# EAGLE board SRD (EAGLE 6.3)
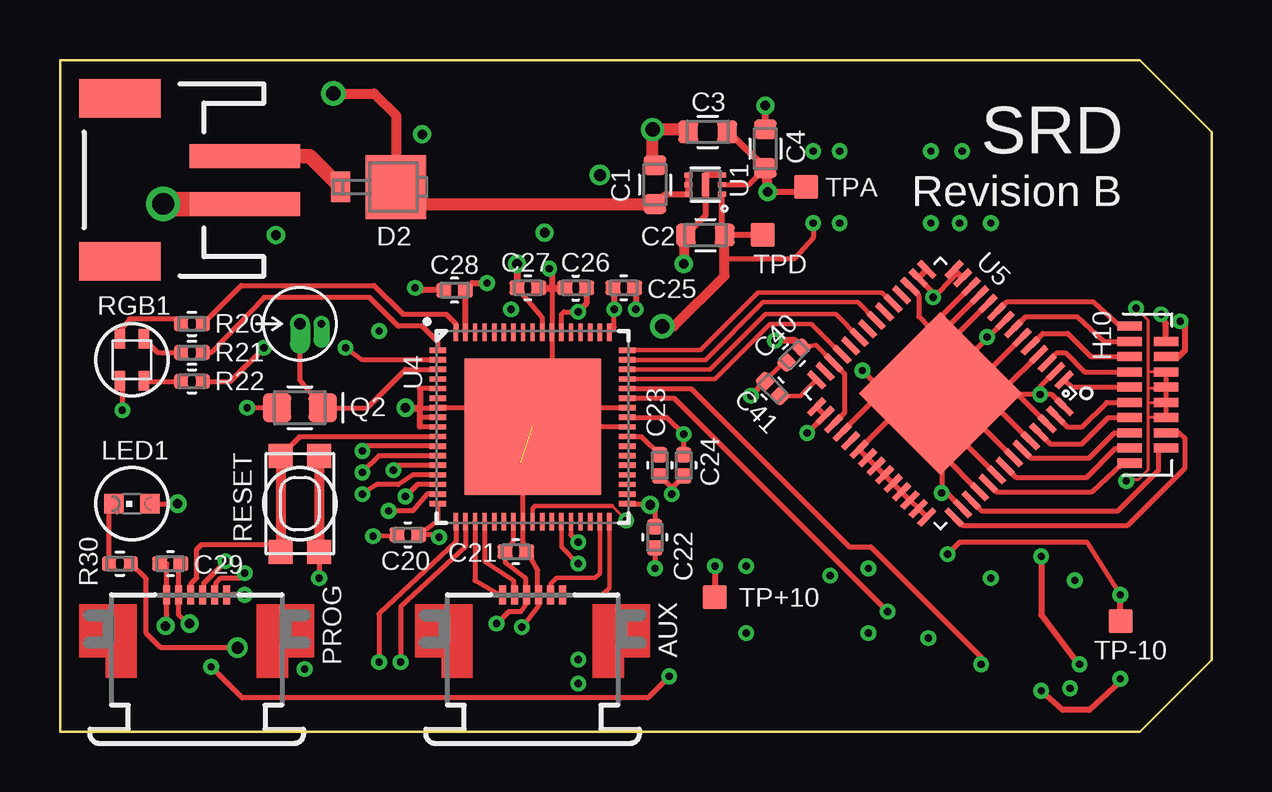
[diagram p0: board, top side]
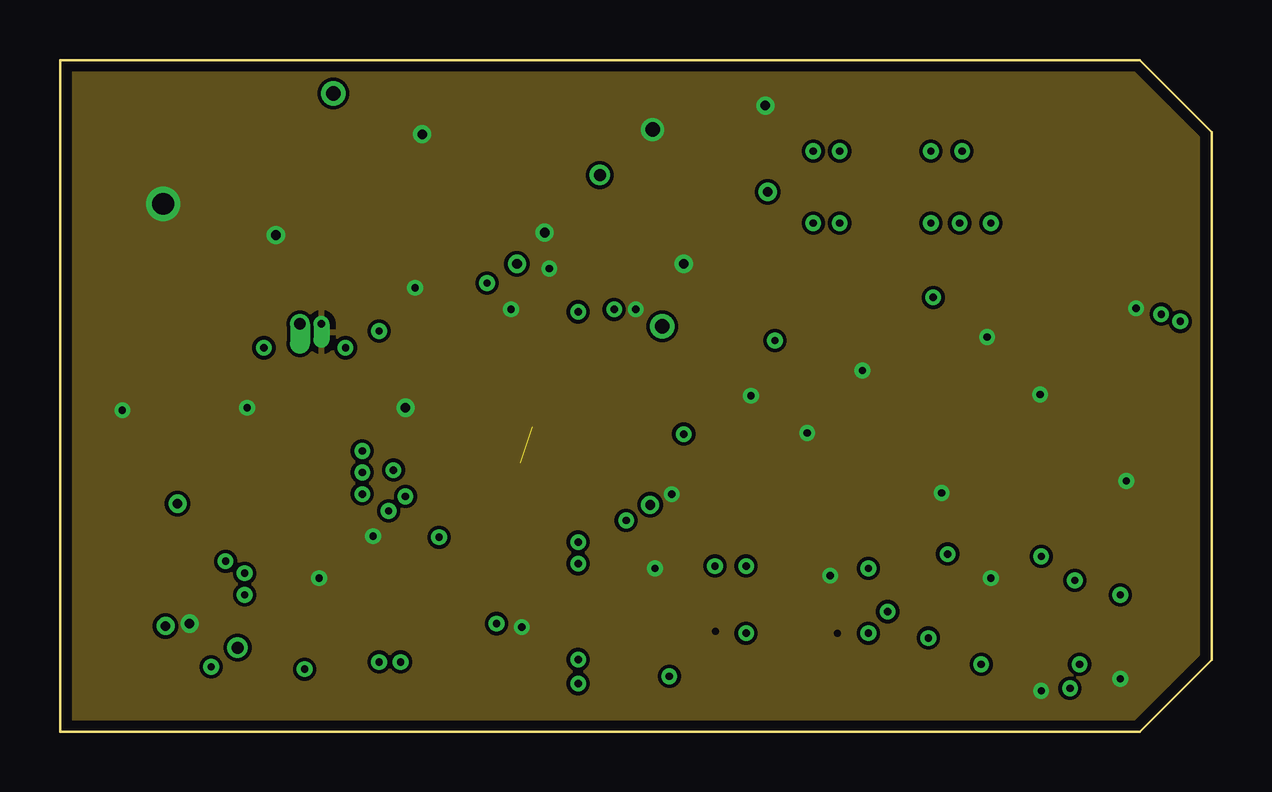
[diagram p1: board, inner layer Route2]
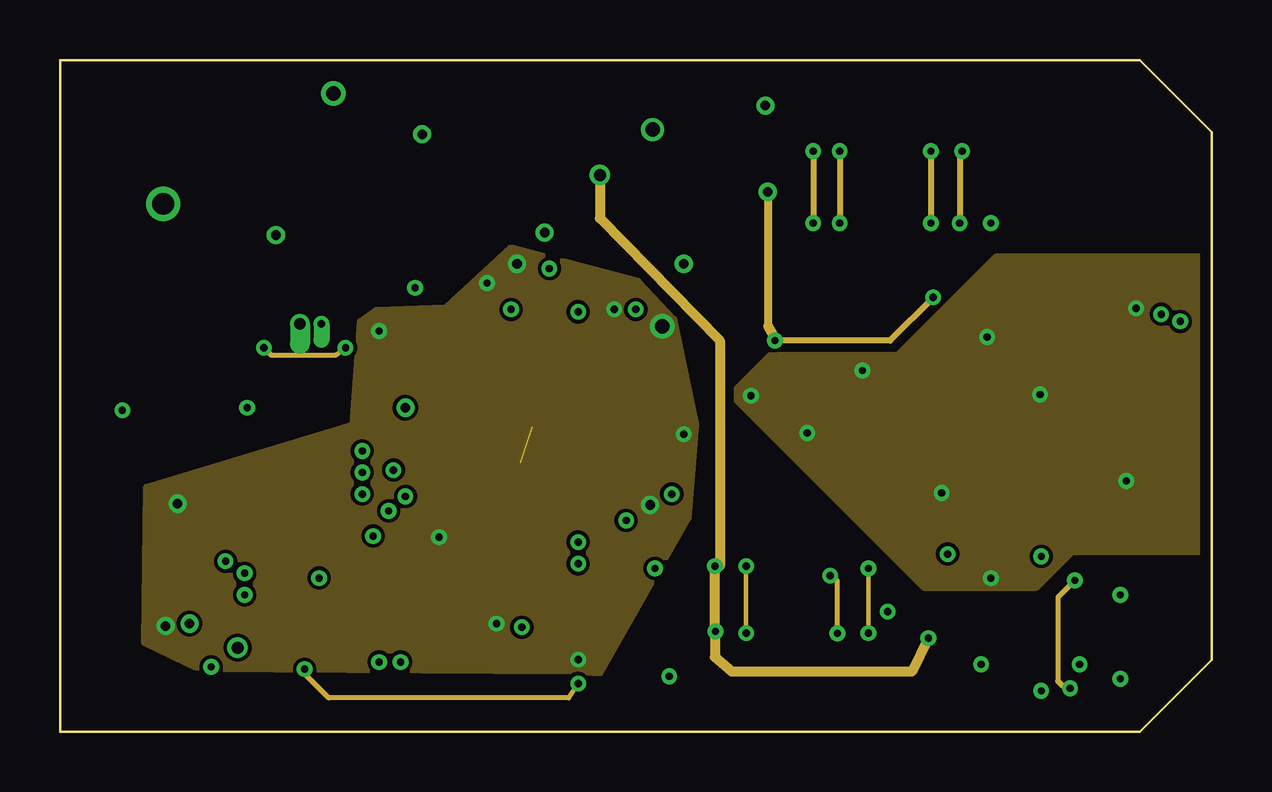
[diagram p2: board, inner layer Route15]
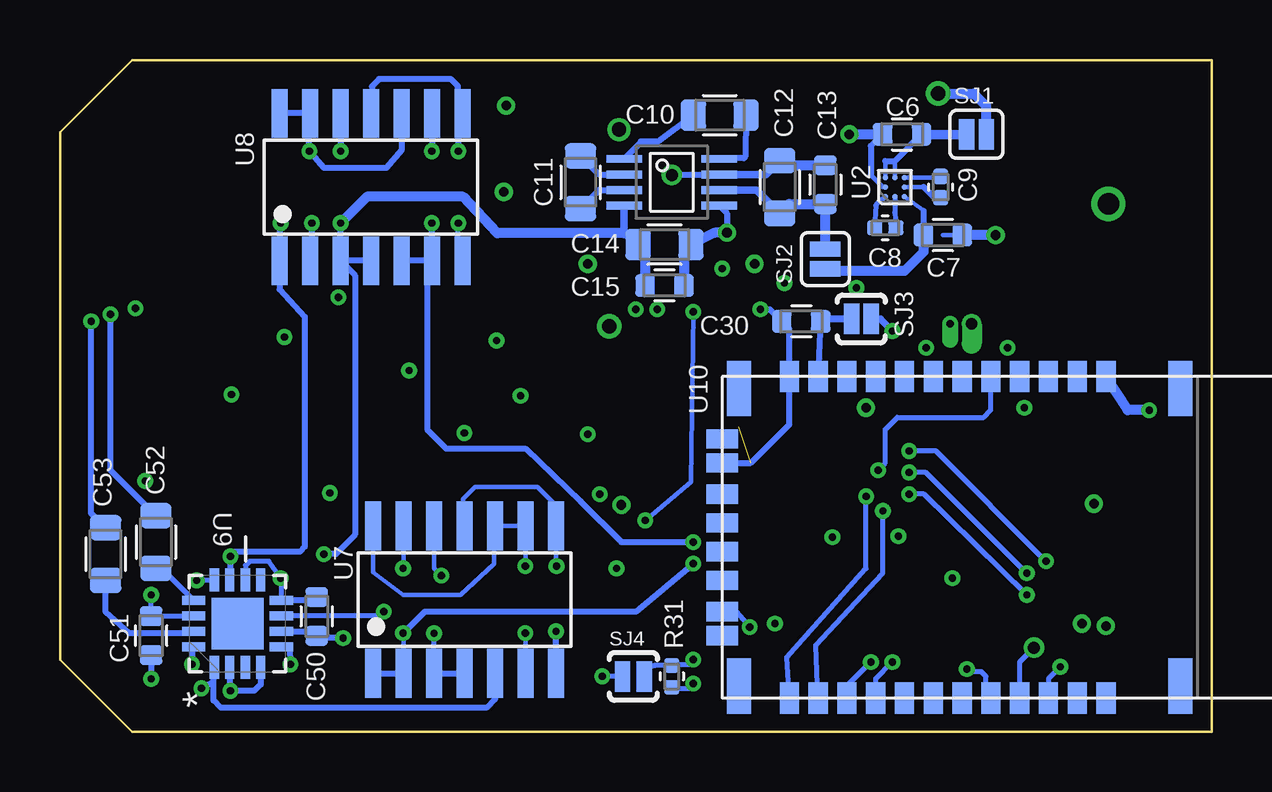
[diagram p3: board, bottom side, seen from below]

Size 48 x 28 mm. Coordinates in mm from the lower left corner, seen from the top.
Outline: 0,0 45,0 48,3 48,25 45,28 0,28 0,0
Copper layers ((1*2)+(15*16)): Top 0.0356mm / dielectric 1.5011mm / Route2 0.0356mm / dielectric 0.1499mm / Route15 0.0356mm / dielectric 0.2007mm / Bottom 0.0356mm
Design rules "LaenPCBOrder_johnmod": minimum track width 5mil, minimum drill 10mil, track to track 6mil, track to pad 6mil, pad to pad 6mil, via to via 6mil, smd to smd 6mil, copper to edge 17mil, drill to drill 6mil, minimum pad ring 7mil, minimum via ring 7mil, stop-mask expansion 0.04mm, vias tented up to drill 0.8mm, thermal gap 10mil

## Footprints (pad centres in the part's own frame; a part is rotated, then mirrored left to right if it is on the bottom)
52746-6 = smd 0.3 x 0.8: 1 -1.25,0.6; 2 -0.75,0.6; 3 -0.25,0.6; 4 0.25,0.6; 5 0.75,0.6; 6 1.25,0.6
JST-2-SMD = smd 1 x 4.6: 1 -1,-3.7; 2 1,-3.7 | smd 1.6 x 3.4: NC1 -3.4,1.5; NC2 3.4,1.5
CAPC1608X90N = smd 0.81 x 0.93: 1 -0.81,0; 2 0.81,0
CAPC1005X55N = smd 0.64 x 0.63: 1 -0.445,0; 2 0.445,0
CAPC2012X100N = smd 1.05 x 1.3: 1 -1.1,0; 2 1.1,0
DO-216AA = smd 0.8 x 1.27: A 0.7,0 | smd 2.54 x 2.67: C -1.6,0
OMNETCS-18PIN-SMD = smd 1.016 x 0.381: 1 1.524,5.715; 2 1.524,5.08; 3 1.524,4.445; 4 1.524,3.81; 5 1.524,3.175; 6 1.524,2.54; 7 1.524,1.905; 8 1.524,1.27; 9 1.524,0.635; 10 1.524,0; 11 0,0.635; 12 0,1.27; 13 0,1.905; 14 0,2.54; 15 0,3.175; 16 0,3.81; 17 0,4.445; 18 0,5.08
CHIPLED_0603 = smd 0.8 x 0.8: A 0,-0.75; C 0,0.75
MTD8000M3B-T = drill 0.47 pad 0.79 offset: C 0,0 | drill 0.32 pad 0.64 offset: E -0.9,0
OP501 = smd 1.2 x 1.2: C -0.955,0; E 0.955,0
RESC1005X35N = smd 0.59 x 0.6: 1 -0.455,0; 2 0.455,0
LED_RGB = smd 0.8 x 0.5: P$1 0.875,-0.5; P$2 -0.875,-0.5; P$3 -0.875,0.5; P$4 0.875,0.5
SJ_2S = smd 0.635 x 1.27: 1 -0.412,0; 2 0.412,0
SJ_2S-NOTRACE = smd 0.635 x 1.27: 1 -0.401,0; 2 0.413,0
SJ_2S-NO = smd 0.635 x 1.27: 1 -0.45,0; 2 0.45,0
KMR2 = smd 1 x 1: 1 2,0.8; 2 2,-0.8; 3 -2,0.8; 4 -2,-0.8
PAD1MMX1MM = smd 1 x 1: P$1 0,0
THIN_DFN = smd 0.35 x 0.18: P$1 -0.7,0.4; P$2 -0.7,0; P$3 -0.7,-0.4; P$4 0.7,-0.4; P$5 0.7,0; P$6 0.7,0.4 | smd 0.3 x 0.94: P$7 0,0
BGA9C40P3X3_121X121X63B27N = smd 0.22 x 0.22: A1 -0.4,-0.4; A2 -0.4,0; A3 -0.4,0.4; B1 0,-0.4; B3 0,0.4; C1 0.4,-0.4; C2 0.4,0; C3 0.4,0.4
UMAX8 = smd 1.5 x 0.3: P$1 -1.98,0.975; P$2 -1.98,0.325; P$3 -1.98,-0.325; P$4 -1.98,-0.975; P$5 1.98,-0.975; P$6 1.98,-0.325; P$7 1.98,0.325; P$8 1.98,0.975
QFN68_8MM_0.4PITCH = smd 0.7 x 0.2: P$1 -3.95,3.2; P$2 -3.95,2.8; P$3 -3.95,2.4; P$4 -3.95,2; P$5 -3.95,1.6; P$6 -3.95,1.2; P$7 -3.95,0.8; P$8 -3.95,0.4; P$9 -3.95,0; P$10 -3.95,-0.4; P$11 -3.95,-0.8; P$12 -3.95,-1.2; P$13 -3.95,-1.6; P$14 -3.95,-2; P$15 -3.95,-2.4; P$16 -3.95,-2.8; P$17 -3.95,-3.2; P$35 3.95,-3.2; P$36 3.95,-2.8; P$37 3.95,-2.4; P$38 3.95,-2; P$39 3.95,-1.6; P$40 3.95,-1.2; P$41 3.95,-0.8; P$42 3.95,-0.4; P$43 3.95,0; P$44 3.95,0.4; P$45 3.95,0.8; P$46 3.95,1.2; P$47 3.95,1.6; P$48 3.95,2; P$49 3.95,2.4; P$50 3.95,2.8; P$51 3.95,3.2 | smd 0.2 x 0.7: P$18 -3.2,-3.95; P$19 -2.8,-3.95; P$20 -2.4,-3.95; P$21 -2,-3.95; P$22 -1.6,-3.95; P$23 -1.2,-3.95; P$24 -0.8,-3.95; P$25 -0.4,-3.95; P$26 0,-3.95; P$27 0.4,-3.95; P$28 0.8,-3.95; P$29 1.2,-3.95; P$30 1.6,-3.95; P$31 2,-3.95; P$32 2.4,-3.95; P$33 2.8,-3.95; P$34 3.2,-3.95; P$52 3.2,3.95; P$53 2.8,3.95; P$54 2.4,3.95; P$55 2,3.95; P$56 1.6,3.95; P$57 1.2,3.95; P$58 0.8,3.95; P$59 0.4,3.95; P$60 0,3.95; P$61 -0.4,3.95; P$62 -0.8,3.95; P$63 -1.2,3.95; P$64 -1.6,3.95; P$65 -2,3.95; P$66 -2.4,3.95; P$67 -2.8,3.95; P$68 -3.2,3.95 | smd 5.7 x 5.7: P$69 0,0
QFN56_8_X_8_LARGE = smd 0.9 x 0.25: 1 -4.05,3.25; 2 -4.05,2.75; 3 -4.05,2.25; 4 -4.05,1.75; 5 -4.05,1.25; 6 -4.05,0.75; 7 -4.05,0.25; 8 -4.05,-0.25; 9 -4.05,-0.75; 10 -4.05,-1.25; 11 -4.05,-1.75; 12 -4.05,-2.25; 13 -4.05,-2.75; 14 -4.05,-3.25; 29 4.05,-3.25; 30 4.05,-2.75; 31 4.05,-2.25; 32 4.05,-1.75; 33 4.05,-1.25; 34 4.05,-0.75; 35 4.05,-0.25; 36 4.05,0.25; 37 4.05,0.75; 38 4.05,1.25; 39 4.05,1.75; 40 4.05,2.25; 41 4.05,2.75; 42 4.05,3.25 | smd 0.25 x 0.9: 15 -3.25,-4.05; 16 -2.75,-4.05; 17 -2.25,-4.05; 18 -1.75,-4.05; 19 -1.25,-4.05; 20 -0.75,-4.05; 21 -0.25,-4.05; 22 0.25,-4.05; 23 0.75,-4.05; 24 1.25,-4.05; 25 1.75,-4.05; 26 2.25,-4.05; 27 2.75,-4.05; 28 3.25,-4.05; 43 3.25,4.05; 44 2.75,4.05; 45 2.25,4.05; 46 1.75,4.05; 47 1.25,4.05; 48 0.75,4.05; 49 0.25,4.05; 50 -0.25,4.05; 51 -0.75,4.05; 52 -1.25,4.05; 53 -1.75,4.05; 54 -2.25,4.05; 55 -2.75,4.05; 56 -3.25,4.05 | smd 4.8 x 4.8: CENTER 0,0
SO14 = smd 2.032 x 0.66: 1 -3.073,4.445; 2 -3.073,3.175; 3 -3.073,1.905; 4 -3.073,0.635; 5 -3.073,-0.635; 6 -3.073,-1.905; 7 -3.073,-3.175; 8 3.073,-3.175; 9 3.073,-1.905; 10 3.073,-0.635; 11 3.073,0.635; 12 3.073,1.905; 13 3.073,3.175; 14 3.073,4.445
QFN65P400X400X100-17N = smd 0.965 x 0.381: 1 -1.829,0.965; 2 -1.829,0.33; 3 -1.829,-0.33; 4 -1.829,-0.965; 9 1.829,-0.965; 10 1.829,-0.33; 11 1.829,0.33; 12 1.829,0.965 | smd 0.381 x 0.965: 5 -0.965,-1.829; 6 -0.33,-1.829; 7 0.33,-1.829; 8 0.965,-1.829; 13 0.965,1.829; 14 0.33,1.829; 15 -0.33,1.829; 16 -0.965,1.829 | smd 2.159 x 2.159: 17 0,0
RN42 = smd 1.3 x 0.8: 1 -6.7,6; 2 -6.7,4.8; 3 -6.7,3.6; 4 -6.7,2.4; 5 -6.7,1.2; 6 -6.7,0; 7 -6.7,-1.2; 8 -6.7,-2.4; 9 -6.7,-3.6; 10 -6.7,-4.8; 11 -6.7,-6; 12 -6.7,-7.2; 13 6.7,-7.2; 14 6.7,-6; 15 6.7,-4.8; 16 6.7,-3.6; 17 6.7,-2.4; 18 6.7,-1.2; 19 6.7,0; 20 6.7,1.2; 21 6.7,2.4; 22 6.7,3.6; 23 6.7,4.8; 24 6.7,6 | smd 0.8 x 1.3: 28 3.1,-10; 29 -3.1,-10; 30 4.1,-10; 31 1.8,-10; 32 0.6,-10; 33 -0.6,-10; 34 -1.8,-10; 35 -4.1,-10 | smd 2.3 x 1: SH1 -6.2,9.1; SH2 -6.2,-9.3; SH3 6.2,-9.3; SH4 6.2,9.1

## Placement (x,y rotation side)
AUX  52746-6  [52746-6]  19.7,5.1 0 top
BAT  M02-JST-2MM-SMT  [JST-2-SMD]  4,23 90 top
C1  1uF  [CAPC1608X90N]  24.8,22.8 90 top
C2  1uF  [CAPC1608X90N]  26.9,20.7 180 top
C3  1uF  [CAPC1608X90N]  27,25 180 top
C4  1uF  [CAPC1608X90N]  29.4,24.3 90 top
C6  2.2uF  [CAPC1608X90N]  12.9,24.9 180 bottom
C7  2.2uF  [CAPC1608X90N]  11.2,20.7 0 bottom
C8  220nF  [CAPC1005X55N]  13.6,21 0 bottom
C9  220nF  [CAPC1005X55N]  11.3,22.7 90 bottom
C10  3.3uF  [CAPC2012X100N]  20.5,25.7 180 bottom
C11  3.3uF  [CAPC2012X100N]  26.3,22.9 90 bottom
C12  3.3uF  [CAPC2012X100N]  18,22.7 90 bottom
C13  1uF  [CAPC1608X90N]  16.1,22.8 90 bottom
C14  3.3uF  [CAPC2012X100N]  22.8,20.3 0 bottom
C15  1uF  [CAPC1608X90N]  22.8,18.6 0 bottom
C20  0.1uF  [CAPC1005X55N]  14.5,8.2 180 top
C21  0.1uF  [CAPC1005X55N]  19,7.5 0 top
C22  0.1uF  [CAPC1005X55N]  24.8,8.1 270 top
C23  1uF  [CAPC1005X55N]  25,11.1 270 top
C24  0.1uF  [CAPC1005X55N]  26,11.1 90 top
C25  0.1uF  [CAPC1005X55N]  23.5,18.5 0 top
C26  0.1uF  [CAPC1005X55N]  21.5,18.5 180 top
C27  1uF  [CAPC1005X55N]  19.5,18.5 0 top
C28  0.1uF  [CAPC1005X55N]  16.45,18.4 0 top
C29  0.1uF  [CAPC1005X55N]  4.6,7 0 top
C30  [CAPC1608X90N]  17.1,17.1 0 bottom
C40  100nF  [CAPC1005X55N]  30.6,15.7 225 top
C41  10nF  [CAPC1005X55N]  29.7,14.3 135 top
C50  0.1uF  [CAPC1608X90N]  37.3,4.8 90 bottom
C51  0.1uF  [CAPC1608X90N]  44.2,4 270 bottom
C52  [CAPC2012X100N]  44,7.9 90 bottom
C53  [CAPC2012X100N]  46.1,7.4 90 bottom
D2  DIODE  [DO-216AA]  12.4,22.7 180 top
H10  A79043-001  [OMNETCS-18PIN-SMD]  46.1,16.9 180 top
LED1  [CHIPLED_0603]  3,9.5 90 top
PROG  52746-6  [52746-6]  5.7,5.1 0 top
Q1  [MTD8000M3B-T]  10,17 180 top
Q2  PHOTOTRANSISTOR_D  [OP501]  10,13.5 180 top
R20  1k  [RESC1005X35N]  5.5,17 180 top
R21  1k  [RESC1005X35N]  5.5,15.8 180 top
R22  1k  [RESC1005X35N]  5.5,14.6 180 top
R30  1k  [RESC1005X35N]  2.5,7 180 top
R31  1k  [RESC1005X35N]  22.5,2.3 90 bottom
RGB1  LED_RGB  [LED_RGB]  3,15.5 270 top
SJ1  SOLDERJUMPERNC  [SJ_2S]  9.8,24.9 0 bottom
SJ2  SOLDERJUMPERNC  [SJ_2S]  16.1,19.7 90 bottom
SJ3  SOLDERJUMPERNC2  [SJ_2S-NOTRACE]  14.6,17.2 0 bottom
SJ4  SOLDERJUMPERNO  [SJ_2S-NO]  24.1,2.3 0 bottom
SW1  SPST_TACT-KMR2  [KMR2]  10,9.5 270 top
TP+10  TEST-POINT  [PAD1MMX1MM]  27.3,5.6 0 top
TP-10  TEST-POINT  [PAD1MMX1MM]  44.2,4.6 0 top
TPA  TEST-POINT  [PAD1MMX1MM]  31.1,22.7 0 top
TPD  TEST-POINT  [PAD1MMX1MM]  29.3,20.7 0 top
U1  MIC5392/3  [THIN_DFN]  26.9,22.8 180 top
U2  AS1302BGA  [BGA9C40P3X3_121X121X63B27N]  13.2,22.7 0 bottom
U3  MAX865  [UMAX8]  22.5,22.9 0 bottom
U4  CY8C3866  [QFN68_8MM_0.4PITCH]  19.7,12.7 0 top
U5  RHD2216_QFN  [QFN56_8_X_8_LARGE]  36.7,14.1 225 top
U7  ALD1105  [SO14]  30.5,5.5 90 bottom
U8  ALD1105  [SO14]  34.4,22.7 90 bottom
U9  DG9409DN-T1-E4  [QFN65P400X400X100-17N]  40.6,4.5 90 bottom
U10  RN42  [RN42]  10.4,8.1 270 bottom

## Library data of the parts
AUX PROG = con-molex; OC_FARNELL: unknown; OC_NEWARK: unknown
BAT = SparkFun-Connectors; PROD_ID: CONN-08352
C1-C4 C6-C15 C20-C30 C40 C41 C50-C53 D2 H10 LED1 Q1 Q2 R20-R22 R30 R31 RGB1 SJ1-SJ4 TP+10 TP-10 TPA TPD U2 U7 U8 U10 = Ramshur
SW1 = _adafruit
U1 U3 U4 = _ramshur
U5 = RHD2000
U9 = DG9409; MPN: DG9409DN-T1-E4; OC_FARNELL: -; OC_NEWARK: 65K2483; PACKAGE: QFN-16; SUPPLIER: VISHAY SILICONIX

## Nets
5VDD: C7.1 SJ2.1 U2.C1
+10VDD: C12.2 C13.2 C50.1 TP+10.P$1 U3.P$7 U7.7 U7.8 U7.11 U9.6
-10VDD: C14.1 C15.1 C51.1 TP-10.P$1 U3.P$4 U8.3 U8.4 U8.12 U9.14
AUX_A1: AUX.5 U4.P$33
AUX_A2: AUX.6 U4.P$34
AUX_D1: AUX.1 U4.P$20
AUX_D2: AUX.2 U4.P$21
AVDD: C3.1 C4.1 C40.1 TPA.P$1 U1.P$2 U5.13 U5.14 U5.15 U5.16 U5.26 U5.31
CH0+: H10.10 U5.9
CH1+: H10.9 U5.7
CH2+: H10.8 U5.5
CH3+: H10.7 U5.3
CH4+: H10.6 U5.1
CH5+: H10.5 U5.55
CH6+: H10.4 U5.53
CH7+: H10.3 U5.51
CH8+: H10.2 U5.49
CH9+: H10.1 U5.47
CH10+: H10.18 U5.45
CH11+: H10.17 U5.43
DVDD: AUX.3 C2.1 C20.1 C21.1 C22.1 C24.2 C25.1 C27.1 C28.2 C29.1 LED1.A PROG.1 R31.2 SJ3.2 SJ4.2 TPD.P$1 U1.P$1 U4.P$17 U4.P$24 U4.P$35 U4.P$44 U4.P$52 U4.P$59 U4.P$67 U8.7 U8.8 U8.11
GND: AUX.4 BAT.1 C1.2 C2.2 C3.2 C4.2 C6.2 C7.2 C14.2 C15.2 C20.2 C21.2 C22.2 C23.2 C24.1 C25.2 C26.2 C27.2 C28.1 C29.2 C30.1 C40.2 C41.2 C50.2 C51.2 H10.13 H10.14 H10.15 H10.16 PROG.2 Q1.E Q2.E RGB1.P$1 SW1.1 SW1.3 U1.P$3 U1.P$7 U2.A2 U3.P$5 U4.P$5 U4.P$7 U4.P$8 U4.P$9 U4.P$25 U4.P$43 U4.P$45 U4.P$58 U4.P$69 U5.2 U5.4 U5.6 U5.8 U5.10 U5.11 U5.12 U5.17 U5.29 U5.30 U5.32 U5.34 U5.35 U5.36 U5.37 U5.38 U5.39 U5.40 U5.41 U5.42 U5.44 U5.46 U5.48 U5.50 U5.52 U5.54 U5.56 U5.CENTER U7.3 U7.4 U7.12 U9.2 U9.4 U9.8 U9.10 U10.1 U10.12 U10.28 U10.29
IDAC1: U4.P$29 U7.1 U7.2 U7.13
IDAC2: U4.P$30 U8.5 U8.6 U8.9
ISTIM+: U7.5 U9.1 U9.12
ISTIM-: U8.1 U9.11 U9.16
LED1: R20.1 U4.P$68
LED2: R21.1 U4.P$1
LED3: R22.1 U4.P$2
MISO: U4.P$48 U5.25
MOSI: U4.P$49 U5.23
N$1: C12.1 C13.1 SJ2.2 U3.P$6
N$2: C41.1 U5.28
N$3: R20.2 RGB1.P$2
N$4: C6.1 SJ1.1 U2.A3 U2.B3
N$5: R21.2 RGB1.P$3
N$6: C52.1 U9.13
N$7: R22.2 RGB1.P$4
N$8: LED1.C R30.2
N$9: C30.2 SJ3.1 U10.11
N$11: U7.6 U7.9 U7.10 U7.14
N$17: C53.1 U9.15
N$30: C23.1 U4.P$42
N$31: U8.2 U8.10 U8.13 U8.14
N$33: C8.1 U2.A1
N$36: C9.2 U2.C3
N$42: C11.1 U3.P$3
N$46: C11.2 U3.P$2
N$47: C10.1 U3.P$8
N$48: C10.2 U3.P$1
N$49: C8.2 U2.B1
N$50: C9.1 U2.C2
PIO2: U10.19
PIO3: R31.1 U10.20
PIO4: SJ4.1 U10.22
PIO5: R30.1 U10.21
RN_RESET: U4.P$13 U10.5
SCLK: U4.P$50 U5.21
SS: U4.P$51 U5.19
STIME1: C52.2 H10.11
STIME2: C53.2 H10.12
STIMSEL0: U4.P$46 U9.7
STIMSEL1: U4.P$47 U9.5
SWDCK: PROG.5 U4.P$12
SWDIO: PROG.4 U4.P$11
SWV: PROG.6 U4.P$14
SYNC: Q1.C Q2.C U4.P$3
UART_CTS: U4.P$18 U10.16
UART_RTS: U4.P$19 U10.15
UART_RX: U4.P$16 U10.14
UART_TX: U4.P$15 U10.13
VBAT: BAT.2 D2.A
VCCD: C26.1 U4.P$26 U4.P$57
VIN: C1.1 D2.C SJ1.2 U1.P$4 U1.P$5 U1.P$6
XRES: PROG.3 SW1.2 SW1.4 U4.P$10

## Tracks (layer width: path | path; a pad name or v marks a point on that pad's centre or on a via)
5VDD
  Bottom 0.178: 12,21.71 U2.C1
  Bottom 0.254: C7.1 12,21.71
  Bottom 0.406: C7.1 12.01,19.99 12.8,19.2 16.09,19.2 SJ2.1
+10VDD  (via drill 0.3, 0.3 layers 15-16, 0.5)
  Top 0.254: v27.3,6.9 TP+10.P$1
  Route15 0.406: v22.5,23.2 22.5,21.4 27.5,16.3 27.5,6.9 v27.3,6.9 27.3,4.2 v27.32,4.17 27.3,4.15 27.3,3.1 28,2.5 35.5,2.5 v36.2,3.9
  Bottom 0.178: U7.11 31.2,8.64 31.2,9.7 30.7,10.2 28.1,10.2 27.32,9.43 U7.8 27.32,6.92 v27.3,6.9
  Bottom 0.254: v22.5,23.2 22.18,23.23 U3.P$7 | U9.6 37.48,4.17 C50.1 | 37.29,3.8 C50.1 | v36.2,3.9 37.21,3.9 C50.1 | U7.7 v27.32,4.17
  Bottom 0.305: C12.2 18.57,23.23 U3.P$7
  Bottom 0.406: C12.2 17.81,23.61 C13.2
-10VDD  (via drill 0.3)
  Top 0.2: v37,7.4 37.5,7.9 42.8,7.9 v44.2,5.7
  Top 0.254: TP-10.P$1 v44.2,5.7
  Route15 0.254: v36.3,24.2 v36.3,21.2
  Bottom 0.2: v44.2,5.7 C51.1 43.92,4.83 U9.14
  Bottom 0.254: U8.4 U8.3 | U8.12 v36.3,24.2 | U8.3 35.7,19.02 35.7,8.2 36.5,7.4 v37,7.4 | U8.3 v36.3,21.2 | U9.14 42.49,4.89
  Bottom 0.305: C14.1 24.32,20.64 24.48,20.78 U3.P$4
  Bottom 0.406: C14.1 23.61,20.01 C15.1 | 35,19.36 U8.4 | 24.48,20.78 29.78,20.78 31.2,22.3 35.2,22.3 v36.3,21.2
AUX_A1
  Top 0.178: U4.P$33 22.5,6.6 22.3,6.4 20.7,6.4 20.45,6.15 AUX.5
AUX_A2
  Top 0.178: U4.P$34 22.9,6 22.6,5.7 AUX.6
AUX_D1
  Top 0.2: U4.P$20 17.3,6.3 18.4,5.65 AUX.1
AUX_D2
  Top 0.2: U4.P$21 17.7,7.1 18.9,6.3 18.9,5.65 AUX.2
AVDD  (via drill 0.3, 0.4)
  Top 0.178: C40.1 31.5,16.11 U5.26
  Top 0.2: U5.16 36.4,18.29 v36.4,18.1 37.27,18.97 U5.14 | U1.P$2 28.71,22.8 C4.1 | U5.26 32.7,14.92 32.7,13.28 U5.31
  Top 0.254: U5.16 U5.15 | U5.13 U5.14 | TPA.P$1 30.9,22.5 v29.5,22.5
  Top 0.3: C4.1 27.89,25 C3.1 | C40.1 30.63,16.3 v29.8,16.3
  Top 0.406: C4.1 v29.5,22.5
  Route15 0.254: v36.4,18.1 34.6,16.3 v29.8,16.3
  Route15 0.3: 29.8,16.4 v29.8,16.3
  Route15 0.34: v29.5,22.5 29.5,16.9
  Route15 0.4: 29.5,16.9 29.8,16.4
CH0+
  Top 0.2: U5.9 39.44,17.9 43.1,17.9 44.2,16.9 H10.10
CH1+
  Top 0.2: U5.7 40.25,17.3 42.4,17.3 43.53,16.27 H10.9
CH2+
  Top 0.2: U5.5 40.97,16.6 42,16.6 42.97,15.63 H10.8
CH3+
  Top 0.2: U5.3 41.58,15.8 41.9,15.8 42.7,14.99 H10.7
CH4+
  Top 0.2: U5.1 42.17,14.36 H10.6
CH5+
  Top 0.2: U5.55 41.99,12.7 42.6,12.7 43.62,13.72 H10.5
CH6+
  Top 0.2: U5.53 41.27,12 42.6,12 43.69,13.09 H10.4
CH7+
  Top 0.2: U5.51 40.46,11.4 42.9,11.4 43.95,12.46 H10.3
CH8+
  Top 0.2: U5.49 39.85,10.6 42.8,10.6 44.02,11.82 H10.2
CH9+
  Top 0.2: U5.47 39.03,10 43,10 44.28,11.19 H10.1
CH10+
  Top 0.2: U5.45 38.42,9.2 44.1,9.2 45.8,10.9 45.8,11.6 45.82,11.82 H10.18
CH11+
  Top 0.2: U5.43 37.6,8.6 44.5,8.6 46.9,11 46.9,12.2 46.65,12.46 H10.17
DVDD  (via drill 0.3, 0.4, 0.6 pad 1.02)
  Top 0.2: U4.P$24 18.9,7.95 C21.1 18.55,7.04 19.4,6.4 19.4,5.65 AUX.3 19.45,5.35 19.2,5 18.7,5 v18.2,4.5 | C20.1 15.75,8.79 U4.P$17 | v4.4,4.4 4.45,4.85 PROG.1 4.45,7 C29.1 | C20.1 15.1,8.04 15.15,8.04 | LED1.A v4.9,9.5 | C27.1 20.1,17.25 U4.P$59 | v15.8,8.1 15.7,8.21 C20.1 | U4.P$52 23.1,16.85 v23.1,17.6 | v31.4,21.2 31.4,20.6 30.6,19.7 27.7,19.7 | C24.2 v26,12.4 25.3,13.1 U4.P$44 | U4.P$35 24.6,9.5 v24.6,9.45 24.8,9.25 C22.1
  Top 0.254: U1.P$1 27.6,20.7 C2.1 TPD.P$1 | U4.P$67 C28.2 17.2,18.7 v17.8,18.7 | C25.1 23.1,18.45 v23.1,17.6
  Top 0.3: v19.05,19.5 C27.1
  Top 0.406: C2.1 27.7,19.7 27.7,19 25.6,16.9 v25.1,16.9
  Route15 0.254: v31.4,24.2 v31.4,21.2
  Bottom 0.2: SJ4.2 arc90 23.2,2.75 R31.2 arc90 22.45,2.8 21.8,2.8 v21.6,3 | 31.4,19.63 v31.4,21.2
  Bottom 0.254: v31.4,24.2 31.4,25.77 U8.8 31.43,26.93 31.7,27.2 34.7,27.2 35,26.9 35,25.74 U8.11 | U8.7 31.4,19.63
  Bottom 0.3: SJ3.2 13.8,17.2 v13.3,16.7
  pour Route15: 24.1,18.8 25.6,17.2 26.5,12.8 26.2,8.9 22.5,2.4 21.2,2.5 5.8,2.6 3.5,3.7 3.6,10.2 12.2,12.8 12.5,17.1 13.2,17.6 16.1,17.7 18.8,20.2
GND  (via drill 0.3, 0.3 layers 15-16, 0.4, 0.6, 0.9 pad 1.42)  (1 unrouted)
  Top 0.127: v44.85,17.65 45.35,17.15 45.35,15 | 45.35,15 45.35,14.3 | 45.35,14.3 45.35,10.9 44.95,10.5 44.5,10.5 | H10.13 45.35,15 | H10.14 46.04,14.3 45.35,14.3 | 46.1,13.7 45.4,13.7 | H10.16 45.4,13.1
  Top 0.178: 21.8,13.4 21.8,12.9 22,12.7 | C40.2 30.18,15.41 C41.2
  Top 0.2: v5.4,4.5 4.95,4.85 PROG.2 4.95,6.8 C29.2 | C20.2 14,8.14 v13.05,8.15 | 15,13.5 U4.P$7 17.4,13.5 | U4.P$8 15,13.1 | U4.P$9 15,12.7 | U4.P$5 15,14.3 | U5.42 U5.41 U5.40 U5.39 U5.38 U5.37 U5.36 U5.35 U5.34 35.04,13.5 35.1,13.5 | U5.29 U5.30 31.16,12.45 v31.15,12.45 | RGB1.P$1 2.6,14.53 v2.6,13.4 | U5.12 36.8,17.38 36.8,17.1 | U5.11 36.9,16.77 36.9,16.4 37.23,16.4 | U5.10 37.23,16.4 | 37.7,15.4 37.7,15.45 U5.8 37.95,15.7 37.7,15.7 37.23,16.17 37.23,16.4 | U5.6 38.5,14.84 38.5,14.7 | U5.4 39.38,14.3 | 39.38,14.3 39.2,14.3 | U5.54 39.68,14.3 39.38,14.3 | U5.56 41.35,14.05 v40.85,14.05 | v40.85,14.05 38.9,14.05 38.45,14.05 | U5.52 39.07,13.5 39,13.5 | U5.50 38.1,13.05 | 38.1,13.05 38.1,13.3 | U5.48 37.6,12.14 | 37.6,12.14 37.6,12.9 | U5.46 36.8,11.53 36.8,11.8 36.75,11.75 v36.75,9.95 36.96,9.95 U5.44 | 38.1,13.05 37.73,13.43 37.05,14.1 U5.CENTER | 37.6,12.14 37.6,11.82 | SW1.1 v10.8,6.4 | Q2.E v7.8,13.5 | 20.5,14.8 U4.P$58 20.5,18.5 | 20.5,14.8 20.4,14.8 | U4.P$43 22,12.7 | 19.3,10.7 U4.P$25 19.3,7.9 19.9,6.7 | U4.P$45 21.9,13.5 arc90 21.8,13.4 21.8,14.8 20.5,14.8 | v19.25,4.35 19.95,5.25 AUX.4 19.95,5.95 19.9,6 | C21.2 19.9,6.75 19.9,6.7 | 19.9,5.7 19.9,6 | 19.9,6 19.9,6.7 | U5.17 35.8,18.18 35.8,17.3 36.23,16.88 36.8,16.88 | U5.32 32.6,12.5 34.2,14.1 34.2,14.3 v33.45,15.05 | U5.2 40.85,14.36 v40.85,14.05 | H10.13 H10.14 H10.15 46.1,13.7 H10.16 | C22.2 v24.8,6.8 | C23.2 25.5,10.15 | C24.1 25.5,10.15 | 25.5,10.15 v25.5,9.9
  Top 0.25: 15,12.7 15,13.1 15,13.5 15,14.3
  Top 0.254: U1.P$3 26.9,23.2 U1.P$7 26.9,21.51 C2.2 26,20.61 | C1.2 24.7,23.71 | C3.2 26.09,25.1 | C41.2 29.39,14.59 v28.8,14 | 37.7,15.4 38.26,14.84 38.5,14.84 | 37.73,13.33 38.4,14 38.5,14 38.45,14.05 38.7,14.3 | 37.6,12.9 37.6,13.2 37.73,13.33 | 37.73,13.33 37.73,13.43 | 39,13.5 38.9,13.6 38.9,14.05 | 38.7,14.3 39.2,14.3 | 38.7,14.3 38.5,14.5 38.5,14.7 | 36.9,16.77 36.8,16.88 36.8,17.1 | U5.CENTER 36.1,13.5 35.1,13.5 | C28.1 15.1,18.4 v14.8,18.5 | v20.4,19.3 20.5,19.2 20.5,18.5 | C25.2 24,18.45 v24,17.6 | v44.2,2.2 44.2,2.1 42.9,0.9 41.8,0.9 v40.9,1.7
  Top 0.3: C27.2 20.5,18.5 C26.2 | v14.4,13.5 15,13.5 | C4.2 v29.4,26.1
  Top 0.406: SW1.3 SW1.1 | 26,20.61 v26,19.5
  Top 0.5: 24.7,23.71 v24.7,25.1 26.09,25.1
  Top 1.016: BAT.1 v4.3,22
  Route15 0.2: v32.41,4.09 32.41,6.29 v32.1,6.5
  Bottom 0.178: 14.2,23.2 13.7,22.7 U2.A2 | C7.2 11.19,20.7 | U7.12 32.41,6.8 v32.1,6.5
  Bottom 0.2: U10.28 19.8,5 v19.25,4.35 | U7.3 v32.41,4.09 | U9.8 38.77,6.37 v38.8,6.4 39.3,7.1 40.1,7.1 40.27,6.93 U9.10
  Bottom 0.254: C6.2 14.2,24.41 14.2,23.2 | U7.3 U7.4 | U9.2 40.9,2.64 v40.9,1.7 39.9,1.7 39.63,1.97 U9.4 | C50.2 37.65,5.46 U9.8 | U3.P$5 20.2,21.61 v20.2,20.8 | C51.2 v44.2,2.2 | v18.8,17.6 18.41,17.6 C30.1 17.6,16.79 U10.12 17.6,12.8 19.2,11.2 U10.29
  Bottom 0.406: v15.1,24.9 C6.2 | v9,20.7 C7.2 | C15.2 21.99,20.11 C14.2 20.7,20.8 v20.2,20.8 | v2.6,13.4 3.5,13.4 U10.1
  other vias: 38.65,16.45 44.45,10.45
  pour Route2: 0.2,0.2 47.8,0.2 47.8,27.9 0.2,27.8
  pour Route15: 47.8,19.8 39,19.8 34.9,15.7 29.6,15.7 28.2,14.3 28.2,13.8 36,6 40.7,6 42.2,7.5 47.8,7.5
IDAC1  (via drill 0.3)
  Top 0.178: U4.P$29 20.9,7.7 v21.6,7
  Route15 0.178: v33.7,6.8 v33.7,4.1
  Bottom 0.178: U7.2 33.67,4.08 v33.7,4.1 | U7.13 33.67,6.83 v33.7,6.8
  Bottom 0.254: U7.1 U7.2 | v21.6,7 24,5 32.8,5 v33.7,4.1
IDAC2  (via drill 0.3)
  Top 0.178: U4.P$30 21.3,8.2
  Top 0.2: 21.3,8.2 v21.6,7.9
  Route15 0.254: v32.5,24.2 v32.5,21.2
  Bottom 0.254: U8.6 U8.5 | U8.9 v32.5,24.2 | U8.6 32.7,19.09 32.7,12.6 31.9,11.8 28.6,11.8 26.3,9.6 24.6,7.9 v21.6,7.9 | U8.6 v32.5,21.2
ISTIM+  (via drill 0.3)
  Route15 0.2: v42.3,6.3 41.6,5.6 41.6,2.1
  Route15 0.254: 41.6,2.1 42,1.7 v42.1,1.8
  Bottom 0.2: U9.12 41.59,6.3 v42.3,6.3
  Bottom 0.254: U7.5 29.86,1.33 30.2,1 41.3,1 41.6,1.3 41.6,2.1 | 41.6,2.1 41.6,2.64 U9.1 | U9.12 41.56,6.37 | v42.1,1.8 41.6,2.1
ISTIM-  (via drill 0.3)
  Top 0.254: v40.9,7.3 40.9,4.86 42.43,2.83 42.47,2.83 v42.5,2.8
  Bottom 0.254: v38.8,21.2 38.84,21.16 U8.1 38.84,18.45 37.8,17.3 37.8,7.7 38,7.5 40.7,7.5 arc-90 v40.9,7.3 40.9,6.36 U9.11 | v42.5,2.8 42.47,3.44 U9.16
LED1
  Top 0.2: R20.1 7.55,18.6 13.1,18.6 14.3,17.4 16.1,17.4 16.5,17 U4.P$68
LED2
  Top 0.2: U4.P$1 15.75,16.25 15.1,16.9 14.1,16.9 12.9,18.1 8.5,18.1 6.3,15.8 R21.1
LED3  (via drill 0.3)
  Top 0.2: U4.P$2 12.6,15.5 v11.9,16 | R22.1 7.1,14.6 v8.5,16
  Route15 0.2: v8.5,16 8.8,15.7 11.5,15.7 v11.9,16
MISO
  Top 0.178: U4.P$48 27.3,14.7 29.6,17 31.32,17 U5.25
MOSI
  Top 0.178: U4.P$49 27.1,15.1 29.4,17.4 32.34,17.4 U5.23
N$1
  Bottom 0.305: C12.1 18.98,22.57 U3.P$6
  Bottom 0.406: C12.1 17.61,21.99 C13.1 SJ2.2
N$2
  Top 0.178: C41.1 30.86,13.98 U5.28
N$3
  Top 0.2: R20.2 4.84,17.2 2.9,17.2 2.5,16.7 RGB1.P$2
N$4
  Bottom 0.178: 13.2,23.79 U2.B3 | U2.A3 13.6,23.79
  Bottom 0.254: C6.1 13.2,23.79 13.6,23.79
  Bottom 0.406: C6.1 10.9,24.89 SJ1.1
N$5
  Top 0.2: RGB1.P$3 4.08,15.8 R21.2
N$6
  Bottom 0.2: U9.13 43.76,6.8
  Bottom 0.406: C52.1 43.76,6.8
N$7
  Top 0.2: RGB1.P$4 3.52,14.6 R22.2
N$8
  Top 0.2: R30.2 2.04,9.29 LED1.C
N$9
  Bottom 0.254: C30.2 U10.11
  Bottom 0.305: SJ3.1 16.3,17.21 C30.2
N$11  (via drill 0.3)
  Route15 0.178: v28.6,6.9 v28.6,4.1
  Bottom 0.178: v28.6,6.9 v28.59,6.91 U7.9 U7.10 29.9,8.54 29.9,7 31.3,5.7 33.7,5.7 34.95,6.64 U7.14 | U7.6 28.59,4.2 v28.6,4.1
N$17
  Bottom 0.254: U9.15 42.6,4.1 45.1,4.1 46.1,5 C53.1
N$30
  Top 0.2: U4.P$42 24.25,12.3 C23.1
N$31  (via drill 0.3)
  Route15 0.254: v37.6,24.2 37.5,24.2 v37.5,21.2
  Bottom 0.254: U8.13 37.8,25.77 | 37.8,25.77 v37.6,24.2 37,23.5 34.4,23.5 33.77,24.23 U8.10 | U8.2 37.5,19.63 v37.5,21.2 | 37.8,25.77 U8.14
N$33
  Bottom 0.2: U2.A1 14,21.95 C8.1
N$36
  Bottom 0.178: U2.C3 11.35,23.1
  Bottom 0.254: 11.35,23.1 C9.2
N$42
  Bottom 0.254: C11.1 25.52,22.57 U3.P$3
N$46
  Bottom 0.254: C11.2 25.52,23.23 U3.P$2
N$47
  Bottom 0.254: C10.1 19.43,23.97 19.5,23.9 20.5,23.9 U3.P$8
N$48
  Bottom 0.254: C10.2 23.07,24.6 23.8,24.6 23.8,24.55 U3.P$1
N$49
  Bottom 0.2: U2.B1 13.2,21.66 C8.2
N$50
  Bottom 0.178: U2.C2 12,22.7
  Bottom 0.254: 12,22.7 11.55,22.25 C9.1
PIO3  (via drill 0.3)
  Route15 0.2: v21.6,2 21.2,1.4 11.2,1.4 10.2,2.4 v10.2,2.6
  Bottom 0.2: R31.1 22.45,1.8 21.8,1.8 v21.6,2 | 9.4,1.9 9.4,2.3 9.6,2.5 10.1,2.5 v10.2,2.6
  Bottom 0.254: 9.4,1.9 U10.20
PIO4  (via drill 0.3)
  Top 0.2: v25.4,2.3 24.5,1.4 7.6,1.4 v6.3,2.7
  Bottom 0.2: v6.3,2.7 6.8,2.2 U10.22 | SJ4.1 v25.4,2.3
PIO5  (via drill 0.5)
  Top 0.2: v7.4,3.5 4.2,3.5 3.6,4.1 3.6,6.36 R30.1
  Bottom 0.2: U10.21 8,2.9 v7.4,3.5
RN_RESET  (via drill 0.3)
  Top 0.2: U4.P$13 14.1,11.1 v13.9,10.9
  Bottom 0.2: v13.9,10.9 13.6,11.2 13.6,12.6 13.1,13.1 9.5,13.1 9.2,13.4 U10.5
SCLK
  Top 0.178: U4.P$50 26.9,15.5 29.3,17.9 33.25,17.9 U5.21
SS
  Top 0.178: U4.P$51 26.7,15.9 29.1,18.3 34.27,18.3 U5.19
STIME1  (via drill 0.3)
  Top 0.254: H10.11 46.1,17 v45.9,17.4
  Bottom 0.254: v45.9,17.4 45.9,10.9 C52.2
STIME2  (via drill 0.3)
  Top 0.127: H10.12 46.07,15.6
  Top 0.254: H10.12 46.63,15.63 46.9,15.9 46.9,17 v46.7,17.1
  Bottom 0.254: C53.2 46.7,9.1 v46.7,17.1
STIMSEL0  (via drill 0.3)
  Top 0.2: U4.P$46 25.6,13.9 v34.5,5
  Bottom 0.2: v34.5,5 34.67,4.83 U9.7
STIMSEL1  (via drill 0.3)
  Top 0.2: U4.P$47 26.3,14.3 32.9,7.7 33.8,7.7 38.4,3.1 v38.4,2.8
  Bottom 0.254: U9.5 38.44,3.54 v38.4,2.8
SWDCK  (via drill 0.3)
  Top 0.2: U4.P$12 13.3,11.5 v12.6,10.8 | PROG.5 arc90 6.5,5.75 6.5,6.2 6.7,6.4 7.5,6.4 v7.7,6.6
  Bottom 0.2: v7.7,6.6 11.9,10.8 v12.6,10.8
SWDIO  (via drill 0.3)
  Top 0.2: U4.P$11 12.8,11.9 v12.6,11.7 | 6,5.75 PROG.4 arc90 6,5.75 | 6,5.75 6,6.2 v6.9,7.1
  Bottom 0.2: v6.9,7.1 11.5,11.7 v12.6,11.7
SWV  (via drill 0.3)
  Top 0.2: U4.P$14 14.7,10.7 14.1,10.3 13.2,10.3 v12.6,9.9 | v7.7,5.7 PROG.6
  Bottom 0.2: v7.7,5.7 12,9.9 v12.6,9.9
SYNC
  Top 0.2: U4.P$3 14.4,15.1 12.8,13.5 Q2.C 10,14.65 Q1.C
UART_CTS  (via drill 0.3)
  Top 0.2: U4.P$18 16.5,7.9 13.3,4.9 v13.3,2.9
  Bottom 0.2: U10.16 14,2.2 v13.3,2.9
UART_RTS  (via drill 0.3)
  Top 0.2: U4.P$19 16.9,7.7 14.2,5.2 v14.2,2.9
  Bottom 0.2: U10.15 15.4,1.9 15.2,1.9 v14.2,2.9
UART_RX  (via drill 0.3)
  Top 0.2: U4.P$16 15.3,9.9 14.7,9.2 v13.7,9.2
  Bottom 0.2: U10.14 16.5,3.6 13.7,6.6 v13.7,9.2
UART_TX  (via drill 0.3)
  Top 0.2: U4.P$15 14.9,10.3 v14.4,9.8
  Bottom 0.2: v14.4,9.8 14.4,6.8 17.7,3.1 U10.13
VBAT
  Top 0.6: BAT.2 10.4,24 D2.A
VCCD  (via drill 0.3)
  Top 0.127: 23,9.4 23.5,8.9
  Top 0.178: U4.P$26 19.7,9.3 19.8,9.4 23,9.4 | v23.6,8.8 23.5,8.9
  Top 0.2: U4.P$57 20.9,17.4 21,17.5 v21.6,17.5
  Top 0.254: C26.1 21.95,17.84 v21.6,17.5
  Bottom 0.178: v21.6,17.5 21.7,10.4 v23.6,8.8
VIN  (via drill 0.6 pad 1.02)
  Top 0.2: D2.C 14,22.59 14.6,21.99
  Top 0.254: C1.1 25.21,22.4 U1.P$6 U1.P$5 U1.P$4
  Top 0.406: v11.4,26.6 13.1,26.6 14,25.7 D2.C
  Top 0.5: 14.6,21.99 C1.1
  Top 0.813: 13.96,21.99 14.6,21.99
  Bottom 0.406: v11.4,26.6 9.9,26.6 9.4,26.1 9.4,24.91 SJ1.2
XRES
  Top 0.2: U4.P$10 10,12.3 SW1.4 | PROG.3 5.45,6.15 5.7,6.4 5.7,7.6 5.9,7.8 8.9,7.8 SW1.2
  Top 0.406: SW1.4 SW1.2

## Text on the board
tPlace: SRD | Revision B
tNames: RESET

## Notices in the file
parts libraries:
SparkFun-Connectors: Licensing: CC v3.0 Share-Alike You are welcome to use this library for commercial purposes.
